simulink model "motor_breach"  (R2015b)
settings: Solver=FixedStepAuto  StartTime=0.0  StopTime=tspan(end)  FixedStep=Ts  RelTol=1e-3
undefined symbols (not defined in the file or in its folder): As, Bs, Cs, Ds

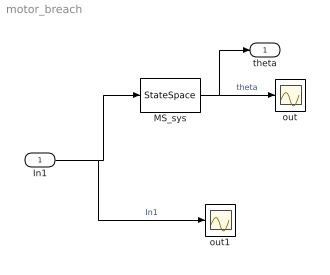
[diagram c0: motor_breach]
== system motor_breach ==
  In1 : Inport
  MS_sys : StateSpace  A=As  B=Bs  C=Cs  D=Ds  X0=0
  out : Scope
  out1 : Scope
  theta : Outport
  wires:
  MS_sys/1 -> theta/1, out/1  "theta"
  In1/1 -> out1/1, MS_sys/1  "In1"
